FUNCTION_BLOCK Example25_stereotypes
VAR_INPUT
	Execute : BOOL;
END_VAR
VAR_OUTPUT
	Done : BOOL;
END_VAR
VAR_IN_OUT
	PM_Controller : PMControllerType;	// the planar motor controller to use
END_VAR
VAR
	PMC_XYMotion1 : PMC_XYMotion;
	cg_array3 : ARRAY[0..2] OF REAL;
	payloadsize_array4 : ARRAY[0..3] OF REAL;
	PMC_MoverStereotype_Define1 : PMC_MoverStereotype_Define;
	PMC_MoverStereotype_ReadDef1 : PMC_MoverStereotype_ReadDef;
	PMC_MoverStereotype_Assign1 : PMC_MoverStereotype_Assign;
	PMC_XYMotion2 : PMC_XYMotion;
	PMC_MoverStereotype_Define2 : PMC_MoverStereotype_Define;
	PMC_MoverStereotype_ReadDef2 : PMC_MoverStereotype_ReadDef;
	PMC_MoverStereotype_Assign2 : PMC_MoverStereotype_Assign;
	PMC_XYMotion3 : PMC_XYMotion;
END_VAR

//4x3 flyways 1 xbot - MoverStereotype Define, Assign, ReadDef

//linear motion to 60,60
PMC_XYMotion1(Execute := Execute,cmdLB := 1,XbotID := 1,Mode := 0,Type_ := 0,PosX := 0.06,PosY := 0.06,EndVel := 0,MaxVel := 1,MaxAcc := 10,PM_Controller := PM_Controller);

//define an unladen, fast stereotype as movertype 0 stereotype 1
cg_array3[0] := 0; cg_array3[1] := 0; cg_array3[2] := 0;
payloadsize_array4[0] := 0; payloadsize_array4[1] := 0; payloadsize_array4[2] := 0; payloadsize_array4[3] := 0;
PMC_MoverStereotype_Define1(Execute := PMC_XYMotion1.Done,MoverType := 0,StereotypeID := 1,PerformanceLevel := 3,Cg := cg_array3,PayloadWeight := 0,PayloadSize := payloadsize_array4,EmergencyStopDecel := 10,PM_Controller := PM_Controller);

//read movertype 0 stereotype 1
PMC_MoverStereotype_ReadDef1(Execute := PMC_MoverStereotype_Define1.Done,MoverType := 0,StereotypeID := 1,PM_Controller := PM_Controller);

//assign movertype 0 stereotype 1 to xbot 1
PMC_MoverStereotype_Assign1(Execute := PMC_MoverStereotype_ReadDef1.Valid,StereotypeID := 1,XbotID := 1,BufferAssign := 0,PM_Controller := PM_Controller);

//linear motion to 900,660
PMC_XYMotion2(Execute := PMC_MoverStereotype_Assign1.Done,cmdLB := 5,XbotID := 1,Mode := 0,Type_ := 0,PosX := 0.9,PosY := 0.66,EndVel := 0,MaxVel := 2,MaxAcc := 20,PM_Controller := PM_Controller);

//define a laden slow stereotype as movertype 0 stereotype 2
cg_array3[0] := 0; cg_array3[1] := 0; cg_array3[2] := 0.03;
payloadsize_array4[0] := 0.12; payloadsize_array4[1] := -0.12; payloadsize_array4[2] := 0.12; payloadsize_array4[3] := -0.12;
PMC_MoverStereotype_Define2(Execute := PMC_XYMotion2.Done,MoverType := 0,StereotypeID := 2,PerformanceLevel := 0,Cg := cg_array3,PayloadWeight := 0.5,PayloadSize := payloadsize_array4,EmergencyStopDecel := 10,PM_Controller := PM_Controller);

//read movertype 0 stereotype 2
PMC_MoverStereotype_ReadDef2(Execute := PMC_MoverStereotype_Define2.Done,MoverType := 0,StereotypeID := 2,PM_Controller := PM_Controller);

//assign movertype 0 stereotype 2 to xbot 1
PMC_MoverStereotype_Assign2(Execute := PMC_MoverStereotype_ReadDef2.Valid,StereotypeID := 2,XbotID := 1,BufferAssign := 0,PM_Controller := PM_Controller);

//linear motion to 60,60
PMC_XYMotion3(Execute := PMC_MoverStereotype_Assign2.Done,cmdLB := 9,XbotID := 1,Mode := 0,Type_ := 0,PosX := 0.06,PosY := 0.06,EndVel := 0,MaxVel := 2,MaxAcc := 20,PM_Controller := PM_Controller);

Done := PMC_XYMotion3.Done;

END_FUNCTION_BLOCK
